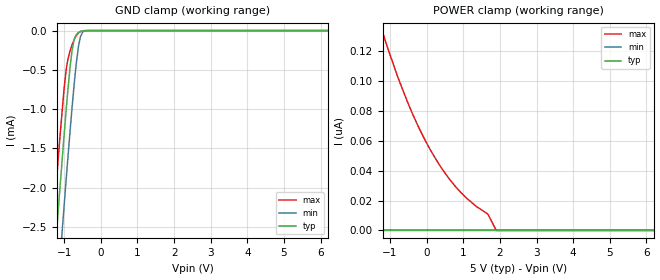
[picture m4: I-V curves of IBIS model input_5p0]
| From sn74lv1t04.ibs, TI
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|   input_5p0 Model
[Model]   input_5p0
Model_type   Input
Vinl = 0.8
Vinh = 2.02
|   typ   min   max
|   (nom PVT)   (fast PVT)   (slow PVT)
C_comp   5.699e-13   5.665e-13   5.768e-13
[Model spec]
|subparameter
Vinl   0.8   0.8   0.8
Vinh   2.02   2.02   2.1
| Where nom  PVT is Nominal Process, 5V, 40C
|   Fast PVT is Strong Process,  5.5V, -40C
|   Slow PVT is Weak Process,   4.5V, 140C
[Voltage Range]   5   4.5   5.5
|Junction Temperature
[Temperature Range]   40   140   -40
[Power Clamp Reference]   5   4.5   5.5
[GND Clamp Reference]   0   0   0
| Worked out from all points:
|   GND clamp passes 1 mA (typ) near -0.95 V on its own axis
[GND Clamp]
|   Voltage   I(typ)   I(min)   I(max)
-5V       -27.41mA   -28.27mA   -26.78mA
-1.535V   -4.632mA   -5.557mA   -3.954mA
-1.265V   -2.919mA   -3.845mA   -2.245mA
-1.155V   -2.24mA    -3.162mA   -1.578mA
-1.121V   -2.029mA   -2.949mA   -1.375mA
-1.007V   -1.35mA    -2.254mA   -756uA
-957.5mV  -1.067mA   -1.957mA   -540.9uA
-790mV    -268uA     -1.002mA   -188.2uA
-671mV    -54.24uA   -419.7uA   -63.93uA
-558.5mV  -11.28uA   -80.02uA   -11.9uA
-297.5mV  -78.67nA   -256.2nA   -52.47nA
10V       0A         0A         0A
[POWER Clamp]
|   Voltage   I(typ)   I(min)   I(max)
-5V       47.4nA     0A         659.7nA
-3.43V    26.17nA    0A         385.5nA
-1.647V   11.35nA    0A         170.9nA
-1.37V    0A         0A         146.5nA
-1.14V    0A         0A         128.1nA
-500mV    0A         0A         84.72nA
-121.5mV  0A         0A         64.33nA
258mV     0A         0A         47.48nA
929mV     0A         0A         25.57nA
1.671V    0A         0A         10.98nA
1.9V      0A         0A         0A
10V       0A         0A         0A
